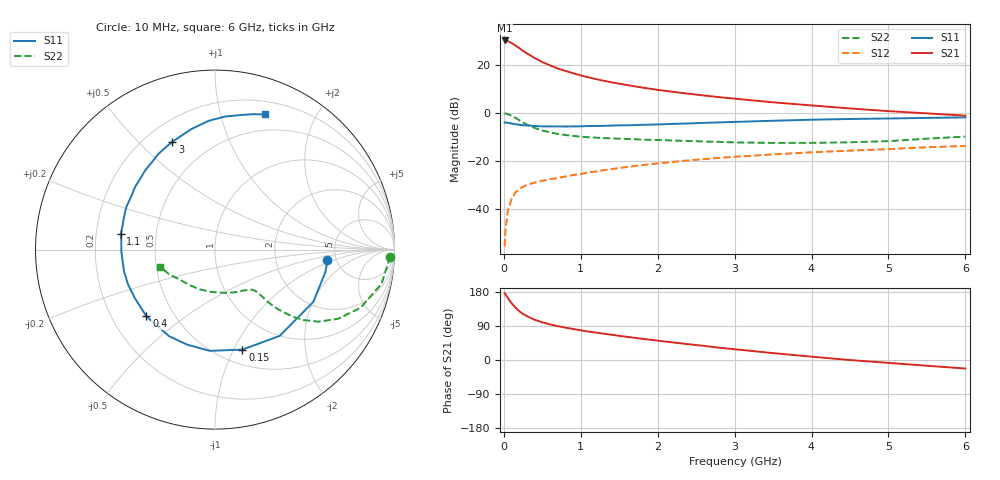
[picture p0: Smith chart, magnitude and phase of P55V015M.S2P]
! SIEMENS Small Signal Semiconductors
! BFP183
! Si NPN RF Bipolar Junction Transistor in SOT143
! VCE = 5 V  IC = 15 mA
! Common Emitter S-Parameters:  March  1996
# GHz  S  MA  R  50
!  f  S11  S21  S12  S22
! GHz  MAG  ANG  MAG  ANG  MAG  ANG  MAG  ANG
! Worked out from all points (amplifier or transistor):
!   36 points, 10 MHz to 6 GHz, reference 50 ohm
!   highest |S21| = 30.0 dB at 10 MHz (marker M1)
!   |S21| within 3 dB of that: start of sweep to 192.7 MHz
!   unconditionally stable (mu >= 1): 980.3 MHz to 5.62 GHz
!   at 250 MHz: K = 0.40, MSG = 28.2 dB, |S12| = -30.7 dB
!   at 1.4 GHz: K = 1.10, MAG = 16.1 dB, |S12| = -23.4 dB
!   at 6 GHz: K = 0.96, MSG = 6.3 dB, |S12| = -13.8 dB
!   S11 on the Smith chart (normalised r, x): 10 MHz: 4.22, -0.84; 150 MHz: 0.65, -1.08; 400 MHz: 0.35, -0.36; 1.1 GHz: 0.31, +0.08; 3 GHz: 0.31, +0.63; 6 GHz: 0.33, +1.39
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0.01  0.6295 -5.5  31.77 176.5  0.0017 86.5  0.9764 -2.3
0.02  0.6278 -11.4  31.64 173.7  0.0034 86.4  0.9668 -4.7
0.05  0.6204 -28.0  30.94 164.1  0.009 79.9  0.9472 -11.6
0.1  0.6008 -53.2  28.07 150.1  0.0161 67.3  0.8734 -21.8
0.15  0.5776 -74.7  25.02 138.3  0.0222 60.2  0.7858 -29.4
0.2  0.5649 -93.0  22.09 128.9  0.0261 54.8  0.7018 -34.9
0.25  0.5519 -106.2  19.27 121.5  0.0291 50.8  0.6306 -38.5
0.3  0.546 -118.0  17.16 115.8  0.0319 48.9  0.5716 -40.8
0.4  0.533 -135.8  13.73 106.2  0.0355 46.5  0.4857 -43.4
0.5  0.5221 -148.7  11.31 99.4  0.0387 45.7  0.4282 -44.5
0.6  0.522 -158.3  9.68 94.0  0.0418 46.0  0.3913 -44.8
0.7  0.5212 -166.5  8.331 89.4  0.0442 47.0  0.3644 -44.9
0.9  0.522 -179.1  6.628 81.9  0.0509 47.8  0.3308 -45.4
1.1  0.532 170.3  5.459 75.0  0.0577 48.7  0.3103 -46.5
1.5  0.5483 154.1  4.019 63.7  0.0714 48.9  0.2898 -50.4
1.8  0.5626 143.3  3.342 55.9  0.0817 48.1  0.2776 -55.0
2.2  0.5882 131.5  2.721 46.3  0.0956 45.9  0.2658 -62.2
3  0.646 111.6  1.964 28.4  0.1219 40.3  0.2429 -80.9
3.5  0.683 101.4  1.65 18.2  0.1368 36.3  0.2368 -94.8
4.5  0.7439 85.5  1.232 -0.1  0.1637 28.0  0.2441 -126.2
5.5  0.7826 74.6  0.972 -15.2  0.1927 20.6  0.2901 -151.6
6  0.8034 69.6  0.873 -22.5  0.2049 16.3  0.321 -162.8
